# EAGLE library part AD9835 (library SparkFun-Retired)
50MHz DDS waveform generator Retired: IC-09105
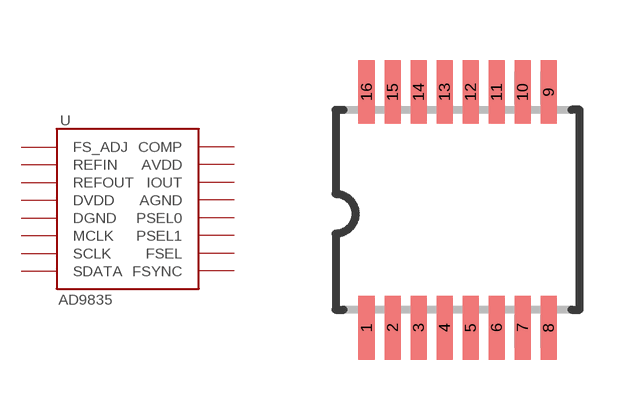
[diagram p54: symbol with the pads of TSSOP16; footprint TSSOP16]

Designator prefix -

## AD9835  [TSSOP16]
1  FS_ADJ
2  REFIN
3  REFOUT
4  DVDD
5  DGND
6  MCLK
7  SCLK
8  SDATA
9  FSYNC
10  FSEL
11  PSEL1
12  PSEL0
13  AGND
14  IOUT
15  AVDD
16  COMP

## Footprint TSSOP16 (pad centres in mm)
TSOP16 thin small outline package
smd 0.4 x 1.6: 1 -2.225,-2.85; 2 -1.575,-2.85; 3 -0.925,-2.85; 4 -0.275,-2.85; 5 0.375,-2.85; 6 1.025,-2.85; 7 1.675,-2.85; 8 2.325,-2.85; 9 2.325,3.05; 10 1.675,3.05; 11 1.025,3.05; 12 0.375,3.05; 13 -0.275,3.05; 14 -0.925,3.05; 15 -1.575,3.05; 16 -2.225,3.05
